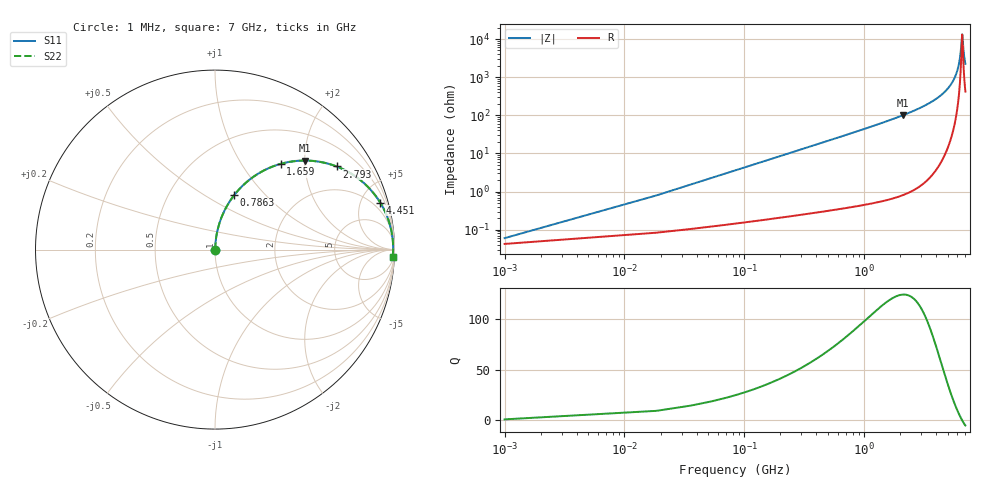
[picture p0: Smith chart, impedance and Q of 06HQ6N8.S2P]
! Coilcraft 0604HQ-6N8 Chip Inductor
! 15 August 2002
# MHZ S MA R 50
!Freq  MagS11  AngS11  MagS21  AngS21  MagS12  AngS12  MagS22  AngS22
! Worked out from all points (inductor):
!   403 points, 1 MHz to 7 GHz, reference 50 ohm
!   read as one part in series: L = 6.8 nH near 35.9 MHz
!   highest Q = 124 at 2.112 GHz (marker M1), where L = 7.58 nH
!   self-resonance near 6.58 GHz
!   S11 on the Smith chart (normalised r, x): 1 MHz: 1.00, +0.00; 786.2 MHz: 1.01, +0.68; 1.659 GHz: 1.01, +1.51; 2.793 GHz: 1.03, +2.91; 4.451 GHz: 1.13, +7.01; 7 GHz: 9, -44
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1  0.0006024 45.1  0.9996 -0.0  0.9996 -0.0  0.0006024 45.1
53.35  0.02279 85.6  0.9985 -1.3  0.9985 -1.3  0.02279 85.6
88.25  0.03766 85.6  0.9978 -2.2  0.9978 -2.2  0.03766 85.6
158.05  0.06731 84.6  0.9959 -3.9  0.9959 -3.9  0.06731 84.6
262.75  0.1115 82.4  0.9915 -6.4  0.9915 -6.4  0.1115 82.4
384.9  0.1624 79.7  0.984 -9.3  0.984 -9.3  0.1624 79.7
786.25  0.3215 70.6  0.9432 -18.8  0.9432 -18.8  0.3215 70.6
1170.15  0.457 62.3  0.8851 -27.2  0.8851 -27.2  0.457 62.3
1658.75  0.6011 52.6  0.7942 -36.9  0.7942 -36.9  0.6011 52.6
2112.45  0.7065 44.6  0.7021 -44.9  0.7021 -44.9  0.7065 44.6
2339.3  0.7499 41.0  0.6555 -48.6  0.6555 -48.6  0.7499 41.0
2793  0.8209 34.3  0.564 -55.2  0.564 -55.2  0.8209 34.3
3508.45  0.8986 25.4  0.4291 -64.0  0.4291 -64.0  0.8986 25.4
4450.75  0.957 15.8  0.2732 -73.1  0.2732 -73.1  0.957 15.8
4677.6  0.9658 13.8  0.2392 -74.9  0.2392 -74.9  0.9658 13.8
5358.15  0.9836 8.3  0.145 -79.4  0.145 -79.4  0.9836 8.3
5846.75  0.99 4.8  0.08386 -80.8  0.08386 -80.8  0.99 4.8
6283  0.9924 1.9  0.03361 -76.0  0.03361 -76.0  0.9924 1.9
6579.65  0.9925 0.0  0.007549 -2.2  0.007549 -2.2  0.9925 0.0
6614.55  0.9924 -0.2  0.008343 24.2  0.008343 24.2  0.9924 -0.2
6806.5  0.9918 -1.4  0.0249 70.1  0.0249 70.1  0.9918 -1.4
7000  0.9908 -2.5  0.04413 76.7  0.04413 76.7  0.9908 -2.5
